[IBIS Ver]   3.2
[File name]   sprm234b.ibs
[File Rev]   3.0
[Date]   Tuesday September 9, 2008
[Source]   File originated at Texas Instruments
[Notes]   Revision History:
   1.0: initial release, 12/21/07
   2.0: 2nd release, 07/31/08
   updated buffer models for
   BI2CSFZP18, BPCI33TPDFZP18
   BPCI33TPUFZP18, IQ33STCKP18PUSR50
   3.0: 3rd release, 09/09/2008
   updated buffer model from 3-state to I/O for
   BSSTL18WGFZ
   THIS IS RELEASE 3.0,THE CONTENTS ARE SUBJECT TO
   CHANGE WITHOUT PRIOR NOTICE,IF NECESSARY.
   Technology type SR50
   version : 3.3V version
   By default all models were done at 3.3V I/O supply besides
   some models associated with DDR interface have 1.8V tips
   Some pins have an input, output and a programmable pull
   associated with them.
   The [model selector] capability of IBIS ver 3.2 has been
   used on this ibis model.
   All the signal names do not contain nomenclature to indicate
   the active level
   For the pins, which are multiplexed with multiple functons,
   normally the reset default function or primary function is
   used for the pin name, for details on multiplexed functions,
   refer to Texas Instruments TMS320DM6437 Digital Media
   Processor data manual (TI literature number SPRS345).
   This file primarily contains the IBIS models for DDR interface
   and some other signals.
   This model passes IBIS syntax checker 4.1.0
   This model succeeds ICX parser syntax check
   IBIS syntax checker reports:
   Errors: 0
   Warnings: 144
   File Passed
   The warnings of "Pulldown Minimum/Typical/Maximum data is
   non-monotonic" are due to the dynamic output control circuit
   or feedback circuit of the buffers.
   The warnings of "Pullup Minimum/Typical/Maximum data is
   non-monotonic" are due to the ESD circuit, and/or damping
   resistor or dynamic output control circuit of the buffers.
   The warnings of "Model XXX: GND/POWER Clamp : Minimum/Typical
   /Maximum value never becomes zero" are caused by the clamp
   leakage.
   The warnings of "Model XXX: The [Falling Waveform]
   with [R_fixture]=XX Ohms and [V_fixture_xx]= XX V ..."
   are caused by either not sufficient simulation time
   for a waveform data or the waveform without the full
   rail-to-rail switching, the IBIS model accuracy has been
   validated against SPICE simulation.
[Disclaimer] Please be aware that in the absence of a written agreement
   Texas Instruments(TI) assumes no liability for:
   (1) The accuracy of the IBIS models provided to your company
   (2) The proper functioning of these Models in your design
   or for any resulting applications;or
   (3)Infringement of patents,copyrights or intellectual
   property rights resulting from your use of these models.
   TI provides IBIS Models as a service to our customers and
   therefore reserves the right to limit distribution of the
   Models.
[Copyright]   Property of Texas Instruments Incorporated.
   Unauthorised reproduction and/or distribution is strictly.
   prohibited.
   This product is protected under copyright law and trade
   secret law as an unpublished work.
   Created 2007,(C) Copyright 2007-2008,
   Texas Instruments Incorporated., All Rights Reserved.
   These commodities are under the U.S.
   Government distribution license control.As such,they are
   not to be re-exported without the prior approval of the
   U.S. Department of Commerce.
[Component]   c64lc_zwt_ddr
[Manufacturer]   Texas Instruments
[Package]
| variable   typ   min   max
R_pkg   3.11358e-01  1.57385e-01  5.62568e-01
L_pkg   3.37358e-09  1.88640e-09  5.29680e-09
C_pkg   1.19001e-12  8.76670e-13  2.13863e-12
[Pin]  signal_name   model_name   R_pin   L_pin   C_pin
M1   CLKOUT   BT3325ESHYPDFZSCP18  2.88371e-01  3.22490e-09  9.97257e-13
T3   PCIEN   IT33SHYPDFZP18  2.25194e-01  2.81970e-09  1.03654e-12
R3   TMS   IT33SHYPUFZP18  1.81087e-01  2.52870e-09  1.03879e-12
P4   TDI   IT33SHYPUFZP18  1.65233e-01  2.71440e-09  1.06601e-12
R2   NTRST   IT33SHYPDFZP18  2.49620e-01  2.93410e-09  1.00161e-12
N4   PORZ   IT33SHYPUFZP18  1.60006e-01  2.60020e-09  1.06735e-12
P3   TDO   OT3350CSFZP18   1.86057e-01  2.90030e-09  1.04506e-12
P2   EMU0   BT3350CSHYPUFZP18  2.66460e-01  2.94120e-09  1.03704e-12
N3   RESETOUTN   OT3350BSFZP18   1.86878e-01  2.77010e-09  9.37047e-13
N2   EMU1   BT3350CSHYPUFZP18  2.15374e-01  2.83270e-09  9.91032e-13
M4   RESETN   IT33SHYPUFZP18  1.65469e-01  2.65260e-09  1.01870e-12
N1   TCK   IQ33STCKP18PUSR50  2.87854e-01  3.19190e-09  9.81015e-13
M3   I2C_DATA   BI2CSFZP18   1.84227e-01  2.57840e-09  9.90638e-13
L4   TINP1L   BT3350CSHYPUFZP18  1.59244e-01  2.46430e-09  1.02831e-12
M2   I2C_CLK   BI2CSFZP18   2.11877e-01  2.92890e-09  1.00477e-12
L3   GIO88   BT3350CSHYPUFZP18  1.75605e-01  2.74180e-09  9.31208e-13
L2   GIO85   BT3350CSHYPUFZP18  2.09892e-01  2.90710e-09  1.00724e-12
K4   TOUT1L   BT3350CSHYPUFZP18  1.57385e-01  1.88640e-09  1.10953e-12
L1   GIO87   BT3350CSHYPUFZP18  2.82240e-01  3.35480e-09  9.95676e-13
K3   GIO86   BT3350CSHYPUFZP18  1.79194e-01  2.78770e-09  8.99479e-13
K2   TINP0L   BT3350CSHYPDFZP18  2.10402e-01  2.74630e-09  1.00599e-12
J4   TOUT0L   BT3350CSHYPDFZP18  1.62125e-01  2.53250e-09  9.91399e-13
J2   CLKR0   BT3350CSHYPDFZP18  2.13435e-01  3.01980e-09  8.93439e-13
J3   DX0   BT3350CSHYPDFZP18  1.75667e-01  2.63700e-09  9.09255e-13
H3   FSX0   BT3350CSHYPDFZP18  2.00924e-01  2.65050e-09  1.05022e-12
H2   FSR1   BT3350CSHYPDFZP18  2.39770e-01  3.02700e-09  9.58053e-13
H4   DR0   BT3350CSHYPDFZP18  1.59212e-01  2.72390e-09  1.03361e-12
H1   CLKX0   BT3350CSHYPDFZP18  2.78104e-01  3.03950e-09  9.52686e-13
G3   DR1   BT3350CSHYPDFZP18  1.89888e-01  2.60520e-09  1.04104e-12
G1   CLKR1   BT3350CSHYPDFZP18  2.87430e-01  3.16730e-09  8.96075e-13
G4   FSR0   BT3350CSHYPDFZP18  1.62402e-01  2.64930e-09  1.00611e-12
G2   DX1   BT3350CSHYPDFZP18  2.32087e-01  2.87720e-09  9.68667e-13
F1   CLKX1   BT3350CSHYPDFZP18  2.90958e-01  2.93810e-09  8.76670e-13
F2   FSX1   BT3350CSHYPDFZP18  2.23429e-01  2.59150e-09  9.40667e-13
F3   GIO4   BT3350CSHYPDFZP18  1.59205e-01  2.59120e-09  9.20981e-13
E1   GIO0   BPCI33TPDFZP18   3.87273e-01  4.13330e-09  1.20137e-12
C1   HCSN   BPCI33TPUFZP18   5.18992e-01  4.97930e-09  1.23935e-12
E2   GIO1   BPCI33TPDFZP18   3.97085e-01  3.81530e-09  1.59967e-12
C2   HINTN   BPCI33TPUFZP18   5.32039e-01  5.29680e-09  1.51749e-12
E3   GIO2   BPCI33TPDFZP18   3.73860e-01  3.52270e-09  1.51366e-12
C3   HDS2N   BPCI33TPUFZP18   3.03316e-01  3.51390e-09  1.59896e-12
E4   GIO3   BPCI33TPDFZP18   2.25063e-01  2.63070e-09  1.46626e-12
C4   HHWIL   BPCI33TPDFZP18   2.61440e-01  3.35420e-09  1.29305e-12
D1   HASN   BPCI33TPUFZP18   4.72701e-01  4.64390e-09  1.35383e-12
C5   HD11   BPCI33TPDFZP18   2.41894e-01  2.72360e-09  1.22744e-12
D2   HRDYN   BPCI33TPUFZP18   4.80973e-01  4.82300e-09  1.59416e-12
B3   HCNTLA   BPCI33TPDFZP18   4.05952e-01  4.02420e-09  1.43354e-12
D3   HCNTLB   BPCI33TPDFZP18   4.47970e-01  4.78070e-09  1.56064e-12
B2   HDS1N   BPCI33TPUFZP18   4.79710e-01  4.43720e-09  1.55456e-12
D4   HD14   BPCI33TPDFZP18   3.84668e-01  3.96350e-09  1.41799e-12
B4   HD13   BPCI33TPDFZP18   3.84608e-01  3.94260e-09  1.31820e-12
D5   HD12   BPCI33TPDFZP18   3.14141e-01  2.96150e-09  1.48582e-12
A3   HRW   BPCI33TPDFZP18   4.80041e-01  4.77230e-09  1.34539e-12
D6   HD06   BPCI33TPDFZP18   2.61328e-01  2.74090e-09  1.39974e-12
B5   HD10   BPCI33TPDFZP18   3.41809e-01  4.02000e-09  1.25183e-12
D7   HD01   BPCI33TPDFZP18   2.21664e-01  3.04990e-09  1.11942e-12
A4   HD15   BPCI33TPDFZP18   4.84786e-01  3.92840e-09  1.34863e-12
C6   HD09   BPCI33TPDFZP18   3.19020e-01  3.52650e-09  1.30846e-12
B6   HD07   BPCI33TPDFZP18   3.41849e-01  3.59230e-09  1.31788e-12
C7   HD04   BPCI33TPDFZP18   2.84362e-01  3.47710e-09  1.27237e-12
A5   HD08   BPCI33TPDFZP18   4.43383e-01  4.01120e-09  1.29621e-12
D8   EM_A_06   BPCI33TPDFZP18   2.75065e-01  3.20810e-09  1.34667e-12
A6   HD05   BPCI33TPDFZP18   4.19458e-01  4.20100e-09  1.22968e-12
B7   HD03   BPCI33TPDFZP18   3.37268e-01  3.41610e-09  1.24779e-12
A7   GIO57  BT3325ETHYPUFZSCP18   3.85151e-01  4.04770e-09  1.17335e-12
C8   HD00   BPCI33TPUFZP18   2.71756e-01  3.07410e-09  1.23205e-12
B8   EM_A_05   BPCI33TPDFZP18   3.12497e-01  3.47520e-09  1.07999e-12
A8   HD02   BPCI33TPDFZP18   3.81009e-01  4.05840e-09  1.07756e-12
D9   EM_A_09   BPCI33TPDFZP18   2.30823e-01  2.33850e-09  1.37410e-12
B9   EM_A_08   BPCI33TPDFZP18   3.43015e-01  3.96650e-09  1.12604e-12
C9   EM_A_07   BPCI33TPDFZP18   3.07716e-01  3.32530e-09  1.25255e-12
A9   EM_A_10   BPCI33TPDFZP18   3.67959e-01  4.09580e-09  1.09155e-12
C10   EM_A_11   BPCI33TPDFZP18   2.53770e-01  2.89280e-09  1.11495e-12
E10   AD26   BPCI33TPDFZP18   3.07231e-01  3.26890e-09  1.36412e-12
B10   CI7   BPCI33TPDFZP18   2.97040e-01  3.58090e-09  1.11309e-12
D10   EM_A_12   BPCI33TPDFZP18   2.42536e-01  2.41830e-09  1.28539e-12
A10   CI6   BPCI33TPDFZP18   3.57840e-01  3.76030e-09  1.12687e-12
C11   CI4   BPCI33TPDFZP18   2.58765e-01  3.02750e-09  1.10900e-12
B11   CI5   BPCI33TPDFZP18   3.19336e-01  3.82120e-09  1.04865e-12
D11   CI2   BPCI33TPDFZP18   2.86822e-01  3.18430e-09  1.41791e-12
A11   CI3   BPCI33TPDFZP18   3.62832e-01  4.13680e-09  1.09368e-12
E11   AD28   BPCI33TPDFZP18   2.18167e-01  2.21350e-09  1.50692e-12
B12   CI1   BPCI33TPDFZP18   3.03341e-01  3.74020e-09  1.06126e-12
E12   AD30   BPCI33TPDFZP18   1.63319e-01  2.19290e-09  1.23267e-12
C12   CI0   BPCI33TPDFZP18   2.63696e-01  3.43490e-09  1.19724e-12
D12   EM_A_21  BT3350CSHYPDFZP18   2.25731e-01  2.89910e-09  1.30733e-12
A12   YI7   BT3350CSHYPDFZP18   3.57745e-01  3.30660e-09  1.09917e-12
A13   VD   BT3350CSHYPDFZP18   3.54741e-01  3.43660e-09  1.03034e-12
B13   YI6   BT3350CSHYPDFZP18   2.88418e-01  3.40630e-09  1.08762e-12
C13   YI5   BT3350CSHYPDFZP18   2.31100e-01  2.97700e-09  1.18679e-12
B14   YI3   BT3350CSHYPDFZP18   2.88111e-01  3.08950e-09  1.06747e-12
A14   PCLK   BT3350CSHYPDFZP18   3.46959e-01  3.68380e-09  1.02475e-12
D13   C_WEN   BT3350CSHYPDFZP18   1.60207e-01  2.20600e-09  1.26165e-12
A15   HD   BT3350CSHYPDFZP18   3.69117e-01  4.14410e-09  1.00348e-12
C14   YI2   BT3350CSHYPDFZP18   2.26066e-01  3.04400e-09  1.18885e-12
B15   YI1   BT3350CSHYPDFZP18   3.02487e-01  3.49540e-09  1.06010e-12
D14   YI4   BT3350CSHYPDFZP18   2.21491e-01  3.05160e-09  1.25521e-12
E14   WRITE_WE BT3350CSHYPUFZP18   1.96623e-01  2.85370e-09  1.30368e-12
C15   YI0   BT3350CSHYPDFZP18   2.42004e-01  2.95610e-09  1.16946e-12
B16   B1   BT3350CSHYPDFZP18   3.30133e-01  3.51610e-09  1.06340e-12
A16   G1   BT3350CSHYPDFZP18   3.88457e-01  3.60760e-09  1.07277e-12
A17   R0   BT3350CSHYPDFZP18   4.10831e-01  3.84020e-09  1.10000e-12
D15   READ_OE  BT3350CSHYPUFZP18   2.28159e-01  3.00560e-09  1.28594e-12
B17   R1   BT3350CSHYPDFZP18   3.49425e-01  3.63070e-09  1.09238e-12
C16   B2   BT3350CSHYPDFZP18   2.76578e-01  2.96490e-09  1.22740e-12
D16   COUT0   BT3350CSHYPDFZP18   2.48607e-01  3.24370e-09  1.26964e-12
D17   COUT2   BT3350CSHYPDFZP18   2.51465e-01  3.23060e-09  1.25714e-12
E16   COUT3   BT3350CSHYPDFZP18   1.86994e-01  2.31600e-09  1.27590e-12
B18   B0   BT3350CSHYPDFZP18   4.03378e-01  3.96850e-09  1.29031e-12
F16   COUT6   BT3350CSHYPDFZP18   1.64337e-01  2.68570e-09  1.14940e-12
C18   LCD_OE   BT3350CSHYPDFZP18   4.21146e-01  3.74780e-09  1.22814e-12
E15   WAIT_BSYN  BT3350CSHYPUFZP18   3.52486e-01  3.21750e-09  1.65847e-12
D18   COUT1   BT3350CSHYPDFZP18   3.36801e-01  3.65590e-09  1.24820e-12
C17   R2   BT3350CSHYPDFZP18   4.58958e-01  4.49520e-09  1.57910e-12
E18   COUT4   BT3350CSHYPDFZP18   2.92483e-01  3.61890e-09  1.34099e-12
F18   YOUT0_BOOTMODE0 BT3350CSHYPDFZP18 2.72734e-01 3.22590e-09 1.33843e-12
G16   YOUT3_BOOTMODE3 BT3350CSHYPDFZP18 2.04484e-01 2.61950e-09 1.27820e-12
C19   G0   BT3350CSHYPDFZP18   5.08093e-01  4.54690e-09  1.37792e-12
E17   COUT5   BT3350CSHYPDFZP18   4.26754e-01  3.96900e-09  1.45462e-12
D19   VCLK   BT3350DSHYPDFZSCP18   4.74130e-01  4.20320e-09  1.30423e-12
F17   COUT7   BT3350CSHYPDFZP18   3.17707e-01  3.47320e-09  1.39000e-12
F15   YOUT1_BOOTMODE1 BT3350CSHYPDFZP18 5.52536e-01 4.58070e-09 1.70444e-12
E19   VSYNC   BT3350CSHYPDFZP18   4.45380e-01  3.61580e-09  1.28626e-12
G17   YOUT4_FASTBOOT  BT3350CSHYPDFZP18 3.21351e-01 3.22390e-09 1.31708e-12
K19   MXI   IOSCHF18SHY   2.88789e-01  3.24080e-09  9.15687e-13
H16   YOUT6_8_16   BT3350CSHYPDFZP18 3.28371e-01 3.64940e-09 1.43701e-12
F19   HSYNC   BT3350CSHYPDFZP18 5.62568e-01  4.78820e-09  1.46104e-12
G15   YOUT2_BOOTMODE2 BT3350CSHYPDFZP18 4.58450e-01  3.77650e-09  2.13863e-12
H15   YOUT7   BT3350CSHYPDFZP18 4.12558e-01  3.38300e-09  1.72240e-12
G19   VPBECLK   BT3350CSHYPDFZP18 5.31976e-01  4.68050e-09  1.42913e-12
H17   YOUT5_LENDIAN   BT3350CSHYPUFZP18 5.00028e-01  4.02790e-09  1.64200e-12
T19   DDR_D_31   BSSTL18WGFZ   3.42526e-01  3.45860e-09  9.40752e-13
U19   DDR_D_30   BSSTL18WGFZ   4.10455e-01  4.00660e-09  1.06342e-12
V18   DDR_D_29   BSSTL18WGFZ   4.00687e-01  3.91430e-09  1.19989e-12
U18   DDR_D_28   BSSTL18WGFZ   3.57509e-01  3.73650e-09  1.16967e-12
T16   DDR_DQM3   BSSTL18WGFZ   2.46413e-01  3.19100e-09  1.23117e-12
U16   DDR_DQS3   BSSTL18WGFZ   3.01572e-01  3.03460e-09  1.17123e-12
W17   DDR_D_27   BSSTL18WGFZ   4.41810e-01  3.87670e-09  1.15697e-12
T18   DDR_D_26   BSSTL18WGFZ   5.40380e-01  4.55740e-09  1.53525e-12
U17   DDR_D_25   BSSTL18WGFZ   4.08028e-01  3.65740e-09  1.43619e-12
V17   DDR_D_24   BSSTL18WGFZ   4.89391e-01  4.13810e-09  1.32028e-12
T17   DDR_D_23   BSSTL18WGFZ   4.69380e-01  3.80540e-09  1.61908e-12
V16   DDR_D_22   BSSTL18WGFZ   3.65710e-01  3.63730e-09  1.15402e-12
W16   DDR_D_21   BSSTL18WGFZ   4.23382e-01  4.08880e-09  1.11923e-12
U15   DDR_D_20   BSSTL18WGFZ   3.09569e-01  3.54810e-09  1.25918e-12
U14   DDR_DQS2   BSSTL18WGFZ   2.76122e-01  3.69810e-09  1.11735e-12
T14   DDR_DQM2   BSSTL18WGFZ   2.22714e-01  3.06870e-09  1.30017e-12
V15   DDR_D_19   BSSTL18WGFZ   3.59823e-01  3.40330e-09  1.20321e-12
W15   DDR_D_18   BSSTL18WGFZ   4.04962e-01  3.73240e-09  1.13874e-12
V14   DDR_D_17   BSSTL18WGFZ   3.20444e-01  3.37300e-09  1.10671e-12
W14   DDR_D_16   BSSTL18WGFZ   3.85041e-01  3.90660e-09  1.04928e-12
W13   DDR_A_00   BSSTL18WGFZ   3.78724e-01  3.89190e-09  1.09655e-12
U13   DDR_A_01   BSSTL18WGFZ   3.04042e-01  3.02430e-09  1.24626e-12
V13   DDR_A_02   BSSTL18WGFZ   3.19306e-01  3.30100e-09  1.09572e-12
U12   DDR_A_03   BSSTL18WGFZ   2.36231e-01  2.90730e-09  1.08519e-12
V12   DDR_A_04   BSSTL18WGFZ   2.89569e-01  3.09430e-09  1.04184e-12
W12   DDR_A_05   BSSTL18WGFZ   3.54550e-01  3.17690e-09  1.02586e-12
W11   DDR_A_06   BSSTL18WGFZ   3.41520e-01  3.96650e-09  9.96671e-13
V11   DDR_A_07   BSSTL18WGFZ   2.76879e-01  3.42150e-09  1.00490e-12
V10   DDR_A_08   BSSTL18WGFZ   2.68477e-01  3.28260e-09  1.03801e-12
U11   DDR_A_09   BSSTL18WGFZ   3.50355e-01  3.80070e-09  1.22405e-12
U10   DDR_A_10   BSSTL18WGFZ   2.17038e-01  2.86130e-09  1.04994e-12
W10   DDR_A_11   BSSTL18WGFZ   3.39278e-01  3.26230e-09  1.00585e-12
W9   DDR_A_12   BSSTL18WGFZ   3.35943e-01  3.13430e-09  1.05996e-12
U8   DDR_BS_00   BSSTL18WGFZ   2.73230e-01  3.19620e-09  1.24720e-12
V9   DDR_BS_01   BSSTL18WGFZ   2.99507e-01  3.57310e-09  1.07291e-12
U9   DDR_BS_02   BSSTL18WGFZ   2.09556e-01  2.84250e-09  1.09796e-12
W8   DDR_CLK0_N   BSSTL18WGFZ   3.26638e-01  3.20780e-09  1.10966e-12
W7   DDR_CLK0   BSSTL18WGFZ   3.22315e-01  3.33030e-09  1.10086e-12
V8   DDR_CKE   BSSTL18WGFZ   2.41690e-01  2.85930e-09  1.20811e-12
T9   DDR_CS_N   BSSTL18WGFZ   1.76590e-01  2.82560e-09  1.19331e-12
T8   DDR_WE_N   BSSTL18WGFZ   1.88661e-01  2.84220e-09  1.16378e-12
U7   DDR_RAS_N   BSSTL18WGFZ   2.39939e-01  3.16740e-09  1.07787e-12
T7   DDR_CAS_N   BSSTL18WGFZ   2.03120e-01  2.76080e-09  1.15544e-12
V7   DDR_D_15   BSSTL18WGFZ   2.93714e-01  3.22850e-09  1.08108e-12
W6   DDR_D_14   BSSTL18WGFZ   3.68509e-01  3.53400e-09  1.02772e-12
V6   DDR_D_13   BSSTL18WGFZ   3.01623e-01  3.29210e-09  1.04182e-12
W5   DDR_D_12   BSSTL18WGFZ   3.88426e-01  3.57200e-09  1.09512e-12
T6   DDR_DQM1   BSSTL18WGFZ   2.17871e-01  2.88480e-09  1.25000e-12
U6   DDR_DQS1   BSSTL18WGFZ   2.67256e-01  3.28360e-09  1.16783e-12
V5   DDR_D_11   BSSTL18WGFZ   3.19565e-01  3.60570e-09  1.06842e-12
U5   DDR_D_10   BSSTL18WGFZ   2.68272e-01  3.23340e-09  1.14279e-12
W4   DDR_D_09   BSSTL18WGFZ   3.97501e-01  3.77730e-09  1.07558e-12
V4   DDR_D_08   BSSTL18WGFZ   3.43317e-01  3.36480e-09  1.08493e-12
W3   DDR_D_07   BSSTL18WGFZ   4.29388e-01  3.75460e-09  1.12682e-12
V3   DDR_D_06   BSSTL18WGFZ   3.71588e-01  3.27970e-09  1.15722e-12
U3   DDR_D_05   BSSTL18WGFZ   3.34523e-01  3.39670e-09  1.22695e-12
V2   DDR_D_04   BSSTL18WGFZ   4.08855e-01  4.01120e-09  1.19626e-12
U4   DDR_DQS0   BSSTL18WGFZ   2.57380e-01  3.03660e-09  1.24997e-12
T4   DDR_DQM0   BSSTL18WGFZ   1.91181e-01  2.91570e-09  1.11355e-12
U2   DDR_D_03   BSSTL18WGFZ   3.54375e-01  3.02860e-09  1.11612e-12
U1   DDR_D_02   BSSTL18WGFZ   3.90588e-01  3.74890e-09  1.04027e-12
T2   DDR_D_01   BSSTL18WGFZ   2.94473e-01  3.14750e-09  1.02013e-12
T1   DDR_D_00   BSSTL18WGFZ   3.40458e-01  3.41600e-09  9.39554e-13
[Model Selector]   IT33SHYPDFZP18
IT33SHYPDFZP18_PD   Cell operated with Pulldown"on"
IT33SHYPDFZP18_Z   Cell operated with Pulldown "off"
[Model Selector]   IT33SHYPUFZP18
IT33SHYPUFZP18_PU   Cell operated with Pullup "on"
IT33SHYPUFZP18_Z   Cell operated with Pullup "off"
[Model Selector]   BT3350CSHYPUFZP18
BT3350CSHYPUFZP18_PU   Cell operated with Pullup "on"
BT3350CSHYPUFZP18_Z   Cell operated with Pullup "off"
[Model Selector]   BT3325ESHYPDFZSCP18
BT3325ESHYPD_PD   Cell operated with Pulldown"on"
BT3325ESHYPD_Z   Cell operated with Pulldown "off"
[Model Selector]   BT3350CSHYPDFZP18
BT3350CSHYPDFZP18_PD   Cell operated with Pulldown"on"
BT3350CSHYPDFZP18_Z   Cell operated with Pulldown "off"
[Model Selector]   BPCI33TPDFZP18
BPCI33TPDFZP18_PD   Cell operated with Pulldown"on"
BPCI33TPDFZP18_Z   Cell operated with Pulldown"off"
[Model Selector]   BPCI33TPUFZP18
BPCI33TPUFZP18_PU   Cell operated with Pullup"on"
BPCI33TPUFZP18_Z   Cell operated with Pullup"off"
[Model Selector]   BT3325ETHYPUFZSCP18
BT3325ETHYPU_PU   Cell operated with Pullup"on"
BT3325ETHYPU_Z   Cell operated with Pullup"off"
[Model Selector]   BT3350DSHYPDFZSCP18
BT3350DSHYPD_PD   Cell operated with Pulldown"on"
BT3350DSHYPD_Z   Cell operated with Pulldown "off"
[Model Selector]   IQ33STCKP18PUSR50
IQ33STCKP18PUSR50_PU   Cell operated with Pullup"on"
IQ33STCKP18PUSR50_Z   Cell operated with Pullup"off"
| Models and submodels in the file (25): OT3350CSFZP18 (3-state), IQ33STCKP18PUSR50_PU (Input), IQ33STCKP18PUSR50_Z (Input), BSSTL18WGFZ (I/O), IOSCHF18SHY (Input), BT3350DSHYPD_Z (I/O), BT3350DSHYPD_PD (I/O), BT3325ETHYPU_Z (I/O), BT3325ETHYPU_PU (I/O), BPCI33TPUFZP18_PU (I/O), BPCI33TPUFZP18_Z (I/O), BPCI33TPDFZP18_PD (I/O), BPCI33TPDFZP18_Z (I/O), BT3350CSHYPDFZP18_PD (I/O), BT3350CSHYPDFZP18_Z (I/O), BT3325ESHYPD_Z (I/O), BT3325ESHYPD_PD (I/O), BI2CSFZP18 (I/O_open_drain), OT3350BSFZP18 (3-state), BT3350CSHYPUFZP18_PU (I/O), BT3350CSHYPUFZP18_Z (I/O), IT33SHYPUFZP18_PU (Input), IT33SHYPUFZP18_Z (Input), IT33SHYPDFZP18_PD (Input), IT33SHYPDFZP18_Z (Input)
